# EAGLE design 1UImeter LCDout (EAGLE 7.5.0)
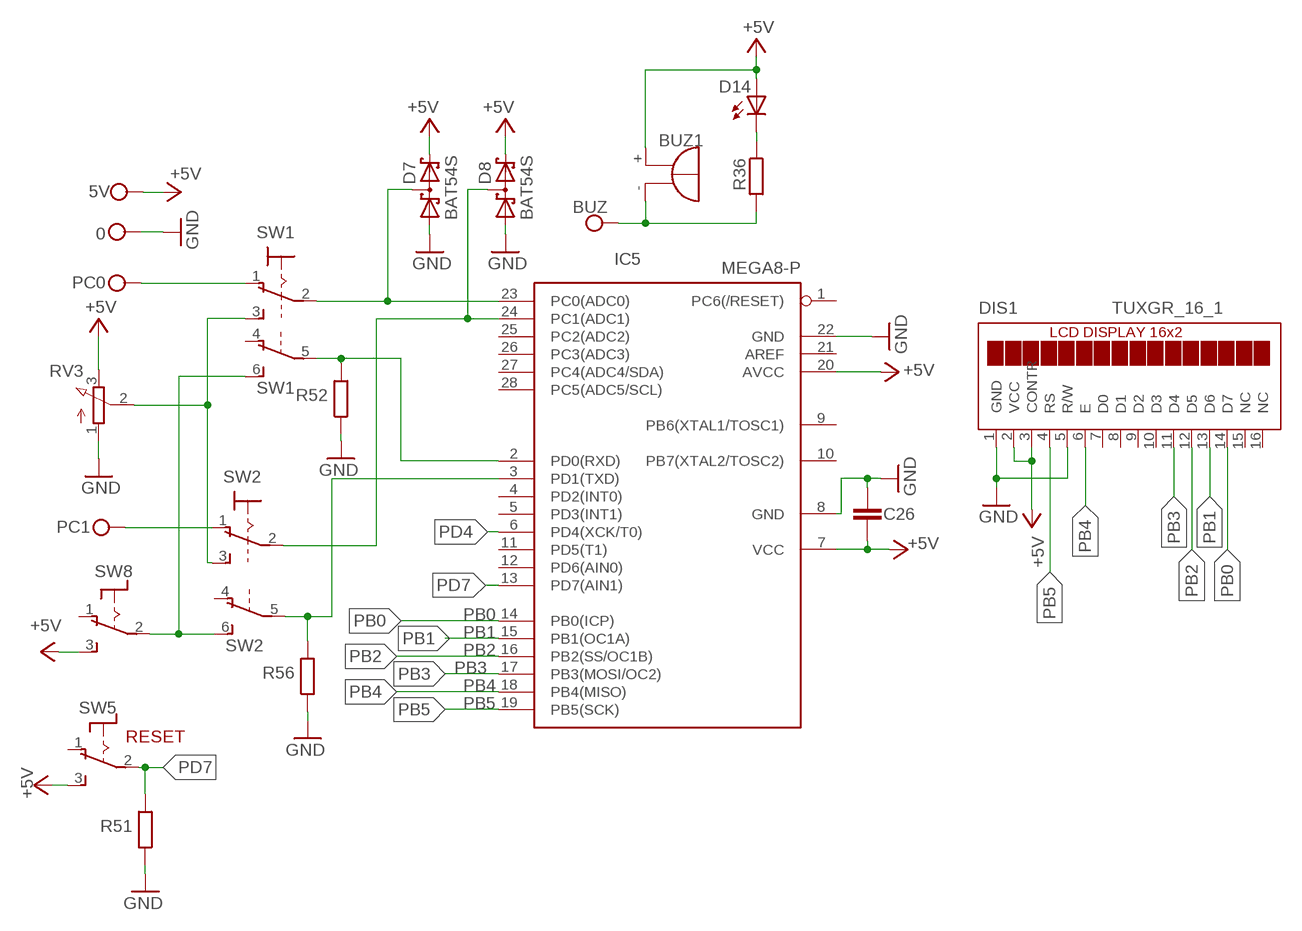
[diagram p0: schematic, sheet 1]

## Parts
0  CONNWIRE  [CONNWIRE]
5V  CONNWIRE  [CONNWIRE]
BUZ  CONNWIRE  [CONNWIRE]
BUZ1  F/HMB  [F/HMB]
C26  C-EUC0805  [C0805]
D7  BAT54S  [SOT23]
D8  BAT54S  [SOT23]
D14  LED3MM  [LED3MM]
DIS1  TUXGR_16_1  [TUXGR_16X1]
IC5  MEGA8-P  [DIL28-3]
PC0  CONNWIRE  [CONNWIRE]
PC1  CONNWIRE  [CONNWIRE]
R36  R-EU_0204/7  [0204/7]
R51  R-EU_0204/7  [0204/7]
R52  R-EU_0204/7  [0204/7]
R56  R-EU_0204/7  [0204/7]
RV3  PTV09A  PV09A  [PTV09]
SW1  320-938  [320-938]
SW2  320-938  [320-938]
SW5  8MS9P1  [8MS9]
SW8  8MS9P1  [8MS9]

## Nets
+5V: 5V.P$1 BUZ1.+ C26.2 D7.2(C2) D8.2(C2) D14.A DIS1.2(VCC) DIS1.3(CONTR) IC5.7(VCC) IC5.20(AVCC) RV3.3(E) SW5.3(S) SW8.3(S)
GND: 0.P$1 C26.1 D7.1(A1) D8.1(A1) DIS1.1(GND) DIS1.5(R/W) IC5.8(GND) IC5.22(GND) R51.1 R52.1 R56.1 RV3.1(A)
N$1: PC1.P$1 SW2.1(1:O)
N$2: PC0.P$1 SW1.1(1:O)
N$4: SW1.6(B:S) SW2.6(B:S) SW8.2(P)
N$5: IC5.2(PD0(RXD)) R52.2 SW1.5(B:P)
N$6: IC5.3(PD1(TXD)) R56.2 SW2.5(B:P)
N$7: D8.3(C1A2) IC5.24(PC1(ADC1)) SW2.2(1:P)
N$19: D14.K(C) R36.1
N$23: BUZ1.- BUZ.P$1 R36.2
PB0: DIS1.14(D7) IC5.14(PB0(ICP))
PB1: DIS1.13(D6) IC5.15(PB1(OC1A))
PB2: DIS1.12(D5) IC5.16(PB2(SS/OC1B))
PB3: DIS1.11(D4) IC5.17(PB3(MOSI/OC2))
PB4: DIS1.6(E) IC5.18(PB4(MISO))
PB5: DIS1.4(RS) IC5.19(PB5(SCK))
PC0: D7.3(C1A2) IC5.23(PC0(ADC0)) SW1.2(1:P)
PD4: IC5.6(PD4(XCK/T0))
PD7: IC5.13(PD7(AIN1)) R51.2 SW5.2(P)
RV3: RV3.2(S) SW1.3(1:S) SW2.3(1:S)
Unconnected: DIS1.7(D0) DIS1.8(D1) DIS1.9(D2) DIS1.10(D3) DIS1.15(NC) DIS1.16(NC) IC5.1(PC6(/RESET)) IC5.4(PD2(INT0)) IC5.5(PD3(INT1)) IC5.9(PB6(XTAL1/TOSC1)) IC5.10(PB7(XTAL2/TOSC2)) IC5.11(PD5(T1)) IC5.12(PD6(AIN0)) IC5.21(AREF) IC5.25(PC2(ADC2)) IC5.26(PC3(ADC3)) IC5.27(PC4(ADC4/SDA)) IC5.28(PC5(ADC5/SCL)) SW1.4(B:O) SW2.4(B:O) SW5.1(O) SW8.1(O)

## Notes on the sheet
- RESET

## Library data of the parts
0 5V BUZ PC0 PC1 = connholes:CONNWIRE
BUZ1 = buzzer:F/HMB: BUZZER; OC_FARNELL: unknown; OC_NEWARK: unknown
C26 = rcl:C-EU: CAPACITOR, European symbol
D7 D8 = diode:BAT54S: Schottky Diodes Pin connection corrected 2011-05-04 Source: Fairchild .. BAT54.pdf
D14 = led:LED: LED
DIS1 = display-lcd:TUXGR_16_1: 1x16 LCD DISPLAY
IC5 = atmel:MEGA8-P: MICROCONTROLLER 8 Kbytes FLASH, 1 kbytes SRAM, 512 bytes EEPROM, USART, 4-channel 10 bit ADC, 2-channel 8 bit ADC Pin compatible with Atmega48, ATMega88, ATMega168 Source: avr.lbr; OC_FARNELL: unknown; OC_NEWARK: unknown
R36 R51 R52 R56 = rcl:R-EU_: RESISTOR, European symbol
RV3 = pot:PV09A
SW1 SW2 = switch:320-938: TOGGLE SWITCH distributor RS Components
SW5 SW8 = switch:8MS9P1

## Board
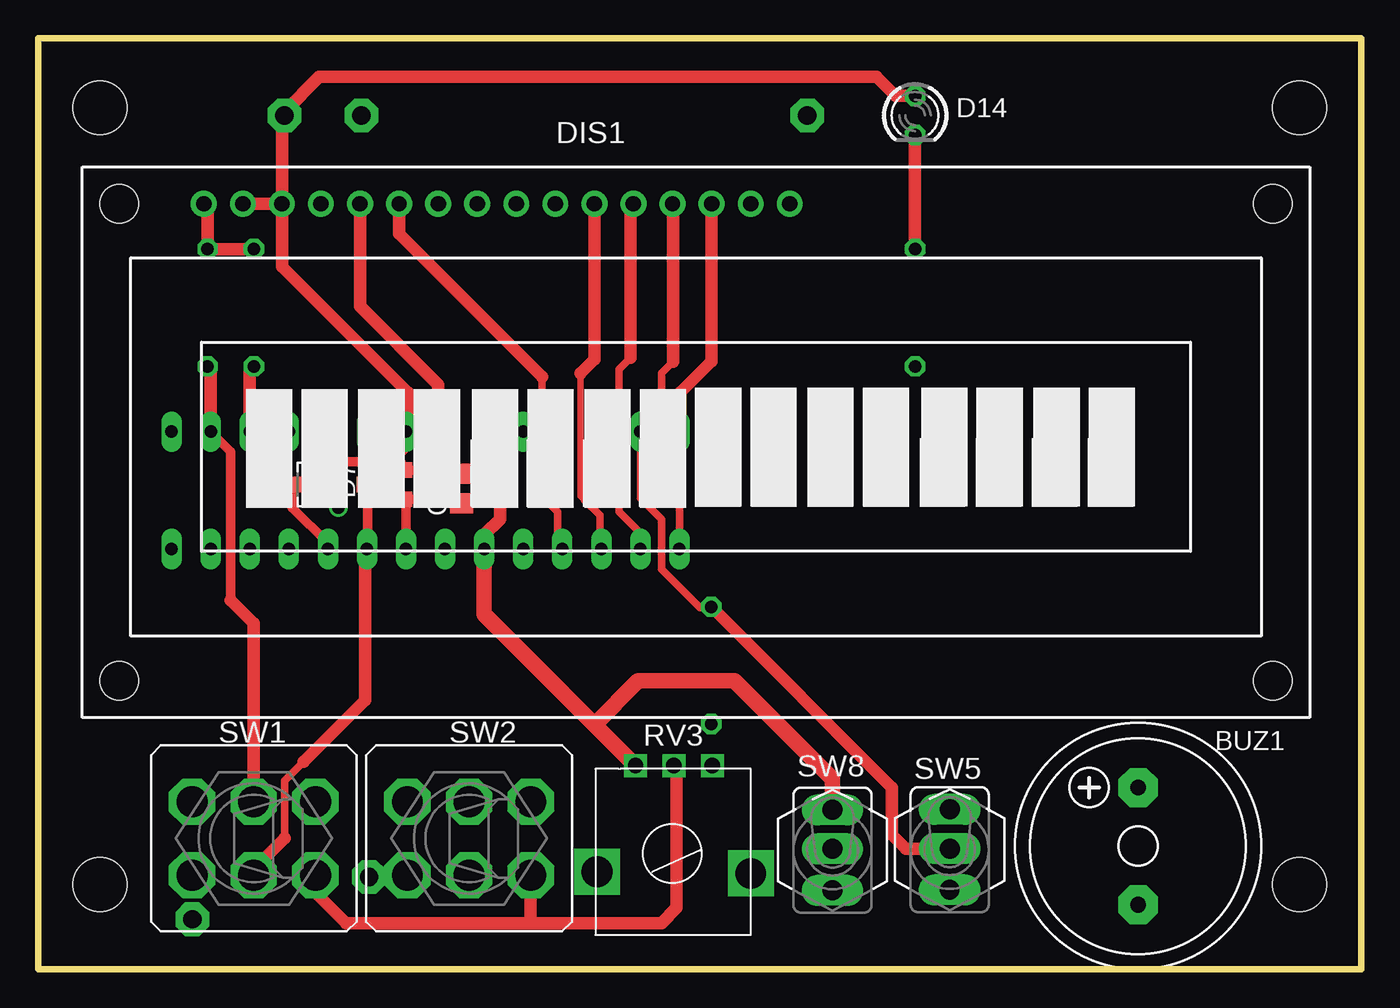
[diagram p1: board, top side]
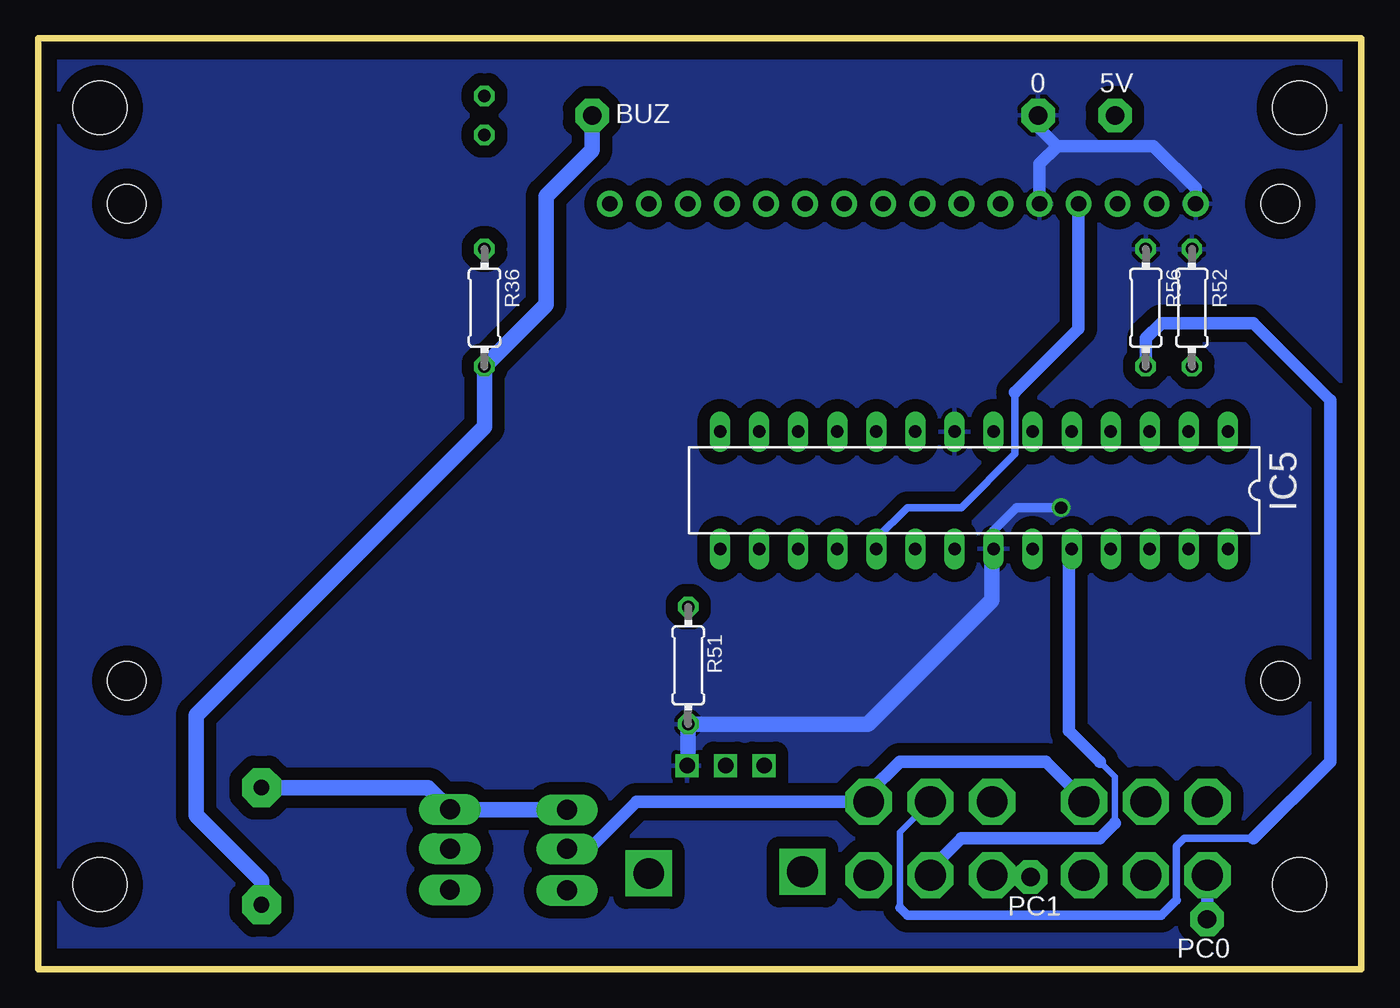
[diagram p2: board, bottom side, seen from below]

Size 86 x 60.5 mm. Coordinates in mm from the lower left corner, seen from the top.
Outline: 0,0 0,60.5 86,60.5 86,0 0,0
Copper layers (1*16): Top 0.035mm / dielectric 1.5mm / Bottom 0.035mm
Design rules "default": minimum track width 10mil, minimum drill 24mil, track to track 8mil, track to pad 8mil, pad to pad 8mil, via to via 8mil, smd to smd 8mil, copper to edge 40mil, drill to drill 8mil, minimum pad ring 10mil, minimum via ring 8mil, stop-mask expansion 4mil, vias tented up to drill 0mil, thermal gap 10mil
Holes 3.5 mm at 4,56 82,56 4,5.5 82,5.5

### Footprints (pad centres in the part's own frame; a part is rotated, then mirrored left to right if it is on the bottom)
CONNWIRE = drill 1.2 pad 2.184 octagon: P$1 0,0
F/HMB = drill 1.016 pad 2.54 octagon: + 3.81,0; - -3.81,0
C0805 = smd 1.3 x 1.5: 1 -0.95,0; 2 0.95,0
SOT23 = smd 1 x 1.4: 1 -0.95,-1.1; 2 0.95,-1.1; 3 0,1.1
LED3MM = drill 0.813 octagon: A -1.27,0; K 1.27,0
TUXGR_16X1 = drill 1 pad 1.676: 1 -0.25,0.26; 2 2.29,0.26; 3 4.83,0.26; 4 7.37,0.26; 5 9.91,0.26; 6 12.45,0.26; 7 14.99,0.26; 8 17.53,0.26; 9 20.07,0.26; 10 22.61,0.26; 11 25.15,0.26; 12 27.69,0.26; 13 30.23,0.26; 14 32.77,0.26; 15 35.31,0.26; 16 37.85,0.26 | hole 2.5: -5.75,-30.74; 69.25,-30.74; -5.75,0.26; 69.25,0.26
DIL28-3 = drill 0.813 long: 1 -16.51,-3.81; 2 -13.97,-3.81; 3 -11.43,-3.81; 4 -8.89,-3.81; 5 -6.35,-3.81; 6 -3.81,-3.81; 7 -1.27,-3.81; 8 1.27,-3.81; 9 3.81,-3.81; 10 6.35,-3.81; 11 8.89,-3.81; 12 11.43,-3.81; 13 13.97,-3.81; 14 16.51,-3.81; 15 16.51,3.81; 16 13.97,3.81; 17 11.43,3.81; 18 8.89,3.81; 19 6.35,3.81; 20 3.81,3.81; 21 1.27,3.81; 22 -1.27,3.81; 23 -3.81,3.81; 24 -6.35,3.81; 25 -8.89,3.81; 26 -11.43,3.81; 27 -13.97,3.81; 28 -16.51,3.81
0204/7 = drill 0.813 octagon: 1 -3.81,0; 2 3.81,0
PTV09 = drill 1 square: 1 -2.5,0; 2 0,0; 3 2.5,0 | drill 2 square: P$4 -5,7; P$5 5,6.9
320-938 = drill 2.007 octagon: 1 -2.388,4.013; 2 -2.388,0; 3 -2.388,-4.013; 4 2.388,4.013; 5 2.388,0; 6 2.388,-4.013
8MS9 = drill 1.295 pad 2 long: 1 -3,5.346 | drill 1.3 pad 2 long: 2 -3,2.654; 3 -3,0.114

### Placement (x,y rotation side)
0  21,55.5 0 bottom
5V  16,55.5 0 bottom
BUZ  50,55.5 0 bottom
BUZ1  71.5,8 90 top
C26  27.5,31.25 90 top
D7  22.5,31.5 90 top
D8  17.5,31.5 90 top
D14  57,55.5 270 top
DIS1  11,49.5 0 top
IC5  25.17,31.13 180 bottom
PC0  10,3.25 0 bottom
PC1  21.5,6 0 bottom
R36  57,43 270 bottom
R51  43.75,19.75 90 bottom
R52  11,43 270 bottom
R56  14,43 270 bottom
RV3  41.32,13.23 180 top
SW1  14,8.5 90 top
SW2  28,8.5 90 top
SW5  56.25,10.5 180 top
SW8  48.63,10.47 180 top

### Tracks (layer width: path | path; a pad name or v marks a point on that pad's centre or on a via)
+5V
  Top 0.61: D8.2 19.45,32.45 20,33 23,33 23.25,33.25 | 23.25,33.25 24,34 24,34.84 IC5.7 | 23.25,33.25 23.6,32.9 D7.2 27.25,32.45 C26.2
  Top 0.813: DIS1.3 15.83,45.67 24,37.5 24,35.04 IC5.7 | D14.A 55.73,56.77 54.5,58 18.25,58 16,55.75 5V.P$1 15.83,55.33 DIS1.3 | DIS1.2 DIS1.3 | IC5.20 28.98,28.23 30,29.25 30,31 28.75,32.25 27.55,32.25 C26.2
  Top 1.016: IC5.20 28.98,23.07 36.15,15.9 | 36.15,15.9 RV3.3 | SW8.3 51.63,12.37 45.25,18.75 39,18.75 36.15,15.9
  Bottom 1.016: SW8.3 59.22,10.36 SW5.3 60.67,11.81 BUZ1.+
GND  (via drill 0.8)
  Top 0.61: C26.1 27.25,30.55 D7.1 23.9,30.25 IC5.22 | D8.1 18.95,30.55 v19.5,30
  Top 0.813: DIS1.1 11,49.51 R52.1 R56.1 | DIS1.5 20.91,43.09 26,38 26,35.38 IC5.8
  Bottom 0.61: v19.5,30 22.4,30 23.9,28.5 IC5.22
  Bottom 0.813: 20.91,55.41 20.91,54.66 19.75,53.5 | 19.75,53.5 13.5,53.5 10.75,50.75 DIS1.1 | DIS1.5 20.91,52.34 19.75,53.5
  Bottom 1.016: RV3.1 43.75,13.3 R51.1 32.06,15.94 24,24 24,27.22 IC5.22
  pour Bottom (isolate 0.813): 0.75,59 85.5,59 85.5,1.5 0.5,1.5 0.5,59
N$1
  Top 0.813: SW2.1 22.11,6.11 22,6 PC1.P$1
N$2
  Bottom 0.813: SW1.1 9.99,3.26 PC0.P$1
N$4
  Bottom 0.813: SW2.6 32.5,10.89 | 32.5,10.89 47.11,10.89 50,8 51.45,8 SW8.2 | SW1.6 18.01,11.01 20.5,13.5 30,13.5 32,11.5 32,11.39 32.5,10.89
N$5
  Top 0.61: 12.5,24 12.5,33.64 IC5.2
  Top 0.813: IC5.2 11.2,38.99 R52.2 | SW1.5 14,22.5 12.5,24
N$6
  Top 0.813: IC5.3 13.74,38.93 R56.2
  Bottom 0.406: 30,4 30,8.89 SW2.5
  Bottom 0.5: 12,4.5 12,8 11.5,8.5 7,8.5
  Bottom 0.61: 30,4 29.5,3.5 13,3.5 12,4.5
  Bottom 0.813: R56.2 14,41 13,42 7,42 2,37 2,13.5 7,8.5
N$7
  Top 0.61: IC5.24 18.82,27.68 16.5,30 16.5,31.4 D8.3
  Bottom 0.406: 16,9.5 16,12.5 17,13.5
  Bottom 0.813: SW2.2 28,6.5 26,8.5 17,8.5 16,9.5 | 17,13.5 19,15.5 19,27.14 IC5.24
N$19
  Top 0.813: R36.1 D14.K
N$23
  Bottom 1.016: BUZ1.- 71.5,5.75 75.75,10 75.75,16.5 57,35.25 R36.2 53,43.19 53,50.25 50,53.25 BUZ.P$1
PB0
  Top 0.813: DIS1.14 43.77,39.52 41.75,37.5 41.75,35.01 IC5.14
PB1
  Top 0.5: IC5.15 41.68,30.82 40.5,32 40.5,38.75 41.25,39.5
  Top 0.813: 41.25,39.5 41.25,49.74 DIS1.13
PB2
  Top 0.5: 38.5,39.75 37.75,39 37.75,29.75 39,28.5 39,27.46 IC5.16
  Top 0.813: 38.5,39.75 38.5,49.57 DIS1.12
PB3
  Top 0.406: 35.25,38.75 35.25,30.75 35.5,30.5
  Top 0.5: 35.5,30.5 36.5,29.5 36.5,27.42 IC5.17
  Top 0.813: DIS1.11 36.15,39.65 35.25,38.75
PB4
  Top 0.5: 32.75,38.5 32.75,30.75 33.75,29.75 33.75,27.63 IC5.18
  Top 0.813: DIS1.6 23.45,47.8 32.75,38.5
PB5
  Bottom 0.5: 22.5,37.5 22.5,33.5 26,30 29.5,30 31.5,28 31.5,27.34 IC5.19
  Bottom 0.813: DIS1.4 18.37,41.63 22.5,37.5
PC0
  Top 0.5: 16,8.5 16,12.25 17.25,13.5
  Top 0.61: D7.3 21.4,27.36 IC5.23
  Top 0.813: 21.5,27.18 IC5.23 21.25,27.21 21.25,17.5 17.25,13.5 | SW1.2 14,6.5 16,8.5
PD7
  Top 0.5: R51.2 43.69,23.5 43,23.5 40.5,26 40.5,29.25 39.14,30.61 IC5.13
  Top 0.813: SW5.2 56.4,7.85 55.5,8.75 55.5,11.81 R51.2
RV3
  Top 0.813: SW1.3 18.01,4.99 20,3 32,3 | 32,3 40.5,3 41.5,4 41.5,13.05 RV3.2 | SW2.3 32.01,3.01 32,3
